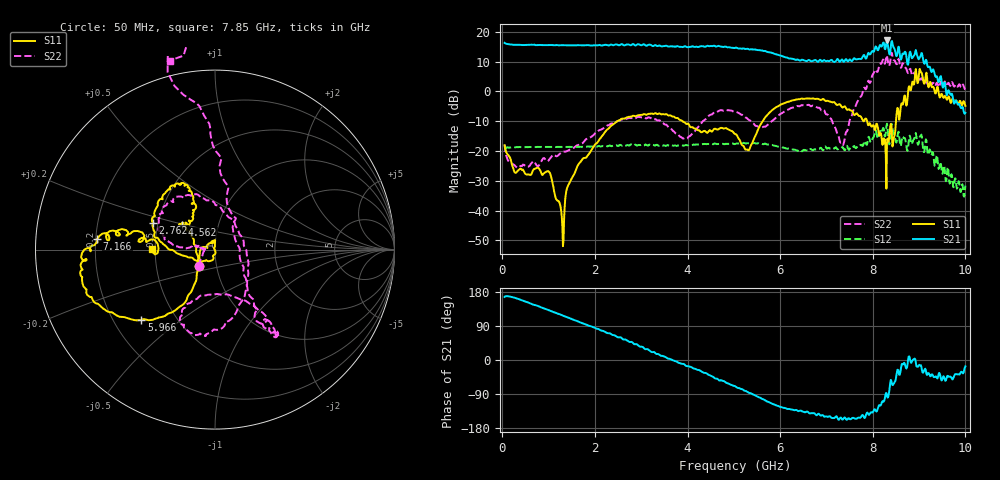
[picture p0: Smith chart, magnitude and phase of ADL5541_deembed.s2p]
! Analog Devices
! ADL5541 RF Gain Block
! These data are intended to be used for performance analysis of the ADL5541.
! These data represent the typical performance of the ADL5541.  No performance guarantees are expressed or implied by
! these data. The test fixture is de-embedded up to the pins of the DUT.
! Created Tue May 22 14:01:24 2007
# hz S db R 50
! 2 Port Network Data from SP1.SP block
! freq  dbS11  angS11  dbS21  angS21  dbS12  angS12  dbS22  angS22
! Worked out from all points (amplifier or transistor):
!   831 points, 50 MHz to 10 GHz, reference 50 ohm
!   highest |S21| = 17.1 dB at 8.306 GHz (marker M1)
!   |S21| within 3 dB of that: start of sweep to 5.328 GHz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
!   unconditionally stable (mu >= 1): start of sweep to 1.985 GHz; 4.013 GHz to 4.269 GHz; 7.064 GHz to 7.578 GHz
!   at 1.706 GHz: K = 1.04, MAG = 15.8 dB, |S12| = -18.6 dB
!   at 5.03 GHz: K = 0.91, MSG = 16.1 dB, |S12| = -17.6 dB
!   at 10 GHz: K = -5.31, MSG = 12.2 dB, |S12| = -31.6 dB
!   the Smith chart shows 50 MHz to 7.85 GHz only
!   S11 on the Smith chart (normalised r, x): 50 MHz: 0.83, -0.15; 2.762 GHz: 0.47, +0.16; 4.562 GHz: 0.67, +0.20; 5.966 GHz: 0.32, -0.37; 7.166 GHz: 0.21, +0.04; 7.85 GHz: 0.48, +0.01
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5e7  -18.11 -134.5  16.29 166.4  -19.15 3.8  -17.89 -134.1
1.298e9  -45.78 138.1  15.51 117.5  -18.62 -38.6  -20.37 167.1
1.718e9  -23.04 -114.9  15.45 97.6  -18.62 -51.6  -17.52 172.9
2.762e9  -8.49 156.6  15.52 47.4  -17.97 -82.9  -8.91 150.7
3.374e9  -7.52 122.2  15.33 15.4  -18.26 -106.5  -9.72 112.4
4.562e9  -12.77 142.7  15.31 -45.2  -17.68 -144.4  -7.14 -84.8
5.03e9  -14.31 145.0  14.63 -69.3  -17.63 -161.1  -6.84 -113.1
5.486e9  -14.22 -122.1  13.95 -95.5  -17.50 179.0  -11.61 -103.8
5.966e9  -4.92 -136.4  12.21 -121.8  -18.56 158.8  -8.07 -54.8
6.686e9  -2.38 -168.8  10.13 -140.2  -19.66 146.6  -4.88 -53.7
7.166e9  -3.61 174.9  9.87 -153.1  -19.18 139.2  -11.51 -48.3
7.85e9  -9.10 179.1  10.99 -146.2  -17.44 147.6  0.69 103.4
8.114e9  -12.38 -159.5  13.79 -125.9  -15.86 173.1  6.98 135.0
8.306e9  -17.50 -78.8  17.10 -93.8  -10.85 -157.8  12.05 163.3
8.342e9  -16.86 -178.5  13.80 -93.0  -16.63 -158.8  8.68 173.9
8.45e9  -15.84 96.7  14.72 -62.9  -14.55 -123.4  10.52 -157.7
8.522e9  -6.44 113.2  11.95 -32.0  -16.56 -83.7  9.15 -132.0
8.642e9  -4.42 99.0  12.66 -10.6  -15.09 -66.0  9.41 -109.7
8.81e9  0.40 87.9  13.35 -1.8  -15.42 -59.4  7.59 -94.3
9.062e9  6.00 14.1  12.80 -26.6  -15.44 -84.4  4.30 -73.0
9.374e9  0.14 -18.3  4.98 -44.4  -21.86 -71.4  2.76 -39.3
1e10  -4.88 -45.9  -7.22 -16.9  -31.62 -38.8  0.64 -13.7
